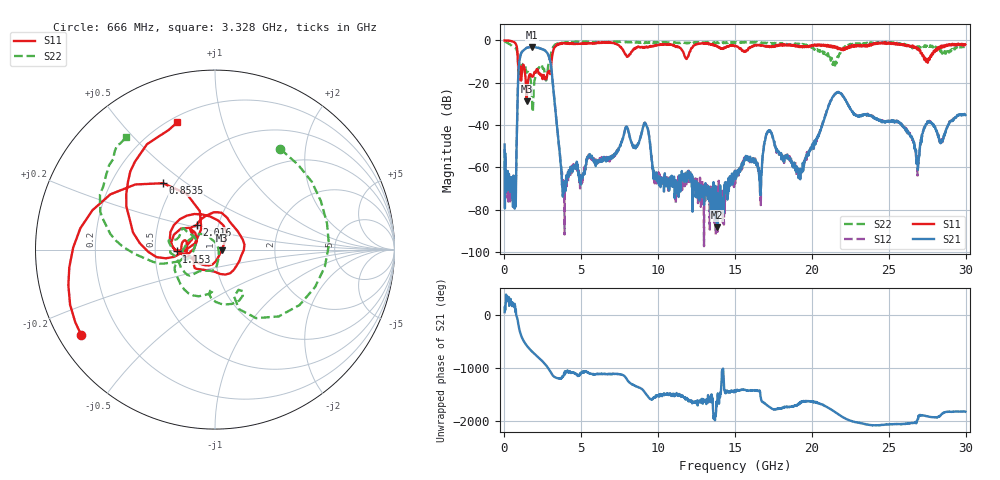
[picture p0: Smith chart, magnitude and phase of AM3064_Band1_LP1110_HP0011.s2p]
# Hz S DB R 50.0
!freq dBS11 angS11 dBS21 angS21 dBS12 angS12 dBS22 angS22
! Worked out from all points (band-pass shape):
!   1600 points, 10 MHz to 29.98 GHz, reference 50 ohm
!   highest |S21| = -3.10 dB at 1.791 GHz (marker M1); lowest = -88.2 dB at 13.84 GHz (marker M2)
!   |S21| within 3 dB of the highest: 1.087 GHz to 2.797 GHz (1.71 GHz wide, 88 % of centre)
!   lowest |S11| = -28.7 dB at 1.435 GHz (marker M3), VSWR 1.08, Z = 53.8 - j0.466 ohm
!   |S11| at or under -10 dB: 876.8 MHz to 3.061 GHz (2.184 GHz wide, 111 % of centre); 27.41291 GHz to 27.43563 GHz (22.73 MHz wide, 0.0829 % of centre); 27.51226 GHz to 27.55153 GHz (39.27 MHz wide, 0.143 % of centre)
!   |S22| runs from -33.8 to -0.4 dB; largest |S21 - S12| = 0.013
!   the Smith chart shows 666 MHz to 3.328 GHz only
!   S11 on the Smith chart (normalised r, x): 666 MHz: 0.07, -0.29; 853.5 MHz: 0.43, +0.41; 1.153 GHz: 0.65, -0.01; 2.016 GHz: 0.79, +0.23; 3.328 GHz: 0.23, +0.72
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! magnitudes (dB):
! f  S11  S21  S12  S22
! 10 MHz  0.0  -49.2  -51.2  -0.4
! 666 MHz  -1.1  -79.5  -65.2  -3.5
! 853.5 MHz  -6.6  -28.2  -28.1  -7.0
! 1.153 GHz  -13.4  -5.3  -5.3  -12.1
! 1.435 GHz  -28.7  -3.6  -3.5  -15.1
! 1.791 GHz  -16.9  -3.1  -3.1  -27.1
! 2.016 GHz  -15.3  -3.3  -3.2  -17.1
! 2.878 GHz  -14.5  -7.3  -7.3  -10.5
! 3.328 GHz  -2.6  -34.0  -34.1  -2.0
! 3.852 GHz  -1.3  -72.0  -70.3  -1.1
! 5.015 GHz  -1.4  -64.3  -67.8  -0.7
! 9.157 GHz  -3.4  -39.2  -39.0  -1.1
! 10 GHz  -2.2  -67.3  -64.4  -0.9
! 13.84 GHz  -2.9  -88.2  -70.3  -1.1
! 15 GHz  -2.6  -63.6  -64.0  -1.3
! 16.62 GHz  -2.1  -68.8  -71.2  -0.9
! 17.2 GHz  -2.7  -43.2  -42.9  -1.1
! 19.99 GHz  -2.8  -50.6  -51.4  -3.1
! 21.64 GHz  -3.3  -24.8  -24.6  -8.6
! 25 GHz  -1.1  -38.0  -38.0  -1.1
! 26.85 GHz  -4.3  -57.1  -60.1  -2.8
! 29.98 GHz  -1.9  -35.3  -35.0  -2.8
